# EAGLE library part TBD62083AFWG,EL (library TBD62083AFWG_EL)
Gate Drivers DMOS Transistor Array 8-CH, 50V/0.5A Source: Datasheet
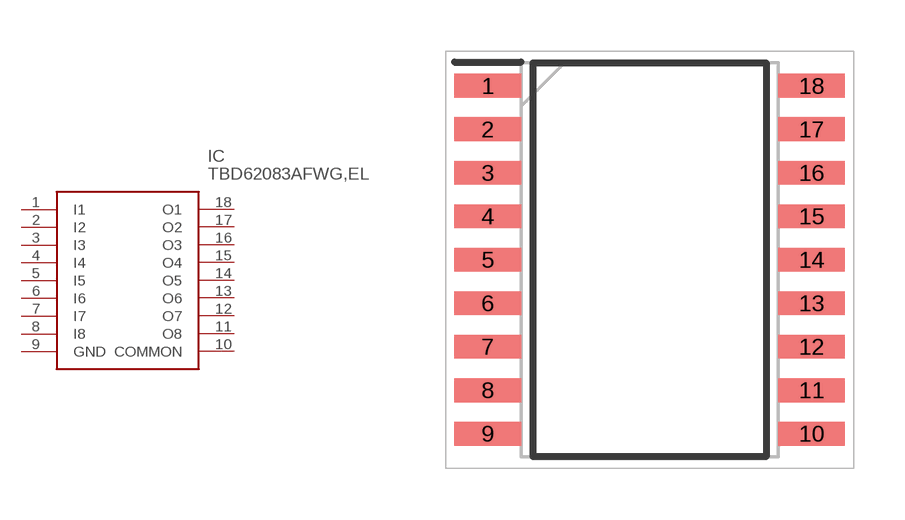
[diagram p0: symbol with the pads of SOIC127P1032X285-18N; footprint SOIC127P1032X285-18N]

Designator prefix IC

## TBD62083AFWG,EL (Description: Gate Drivers DMOS Transistor Array 8-CH, 50V/0.5A; Height: 2.85mm; Manufacturer_Name: Toshiba; Manufacturer_Part_Number: TBD62083AFWG,EL; Mouser_Part_Number: 757-TBD62083AFWGEL; Mouser_Price-Stock: https://www.mouser.co.uk/ProductDetail/Toshiba/TBD62083AFWGEL?qs=fSnNYG2PaKJPpDBB6xK1QA%3D%3D)  [SOIC127P1032X285-18N]
1  I1
2  I2
3  I3
4  I4
5  I5
6  I6
7  I7
8  I8
9  GND
10  COMMON
11  O8
12  O7
13  O6
14  O5
15  O4
16  O3
17  O2
18  O1

## Footprint SOIC127P1032X285-18N (pad centres in mm)
P-SOP18-0812-1.27-001
smd 1.95 x 0.7: 1 -4.725,5.08; 2 -4.725,3.81; 3 -4.725,2.54; 4 -4.725,1.27; 5 -4.725,0; 6 -4.725,-1.27; 7 -4.725,-2.54; 8 -4.725,-3.81; 9 -4.725,-5.08; 10 4.725,-5.08; 11 4.725,-3.81; 12 4.725,-2.54; 13 4.725,-1.27; 14 4.725,0; 15 4.725,1.27; 16 4.725,2.54; 17 4.725,3.81; 18 4.725,5.08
